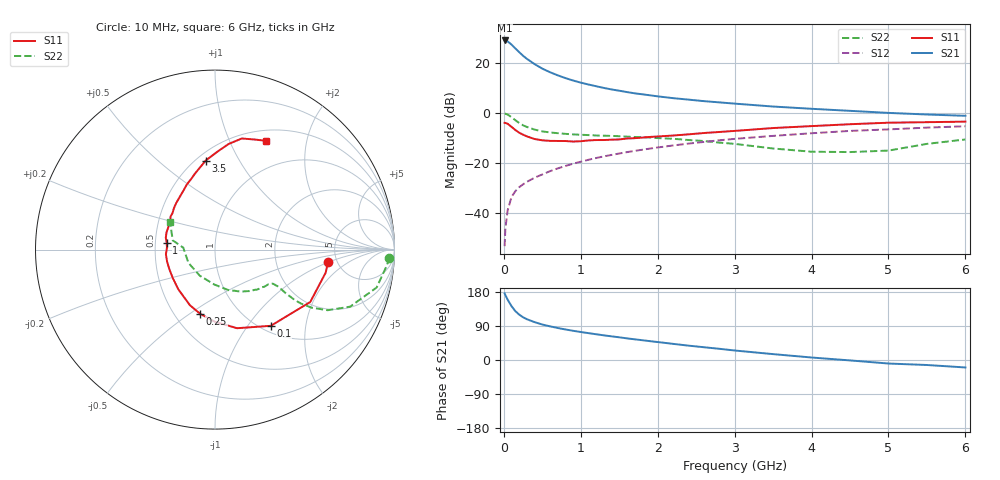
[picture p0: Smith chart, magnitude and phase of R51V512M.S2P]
! SIEMENS Small Signal Semiconductors
! BFR183
! Si NPN RF Bipolar Junction Transistor in SOT23
! VCE = 1.5 V  IC = 12 mA
! Common Emitter S-Parameters:  May  1996
# GHz  S  MA  R  50
!  f  S11  S21  S12  S22
! GHz  MAG  ANG  MAG  ANG  MAG  ANG  MAG  ANG
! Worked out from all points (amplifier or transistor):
!   36 points, 10 MHz to 6 GHz, reference 50 ohm
!   highest |S21| = 28.9 dB at 10 MHz (marker M1)
!   |S21| within 3 dB of that: start of sweep to 143.7 MHz
!   unconditionally stable (mu >= 1): 675.4 MHz to 2.536 GHz
!   at 250 MHz: K = 0.69, MSG = 25.6 dB, |S12| = -28.5 dB
!   at 1.4 GHz: K = 1.06, MAG = 11.6 dB, |S12| = -16.8 dB
!   at 6 GHz: K = 0.91, MSG = 2.1 dB, |S12| = -5.3 dB
!   S11 on the Smith chart (normalised r, x): 10 MHz: 4.22, -0.98; 100 MHz: 1.10, -1.30; 250 MHz: 0.67, -0.55; 1 GHz: 0.57, +0.05; 3.5 GHz: 0.56, +0.73; 6 GHz: 0.63, +1.37
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0.01  0.6338 -6.3  27.78 175.7  0.0022 88.6  0.9732 -2.6
0.02  0.6298 -11.8  27.59 171.2  0.005 80.5  0.9607 -5.4
0.05  0.6057 -28.8  26.59 159.0  0.0115 77.0  0.9251 -13.2
0.1  0.5263 -53.8  22.97 142.1  0.0211 70.2  0.8171 -22.9
0.15  0.455 -74.3  19.24 128.8  0.0275 65.3  0.7124 -28.3
0.2  0.402 -90.0  16.22 119.7  0.033 63.5  0.6283 -31.0
0.25  0.3676 -102.9  13.76 112.8  0.0376 62.4  0.5652 -32.1
0.3  0.3398 -114.3  11.94 107.6  0.0422 63.3  0.5237 -32.3
0.4  0.3013 -132.6  9.375 99.9  0.051 64.0  0.4641 -31.7
0.5  0.2836 -146.0  7.627 93.6  0.0592 65.1  0.4272 -30.8
0.6  0.2768 -156.5  6.464 88.8  0.0688 65.9  0.4073 -30.4
0.7  0.2753 -166.2  5.607 84.5  0.078 66.1  0.3935 -30.4
0.8  0.2746 -174.7  4.937 80.6  0.0874 66.2  0.3819 -30.4
1  0.272 171.7  4.007 73.9  0.1061 66.0  0.3667 -31.3
1.1  0.2819 166.5  3.678 70.9  0.1161 65.9  0.3604 -32.4
1.3  0.2874 156.0  3.142 65.1  0.1357 64.5  0.3505 -34.3
1.6  0.3083 143.5  2.599 57.1  0.1649 62.2  0.3358 -38.6
2.2  0.3533 123.8  1.966 42.6  0.224 56.7  0.3043 -49.4
3.5  0.4985 96.0  1.338 15.5  0.3476 40.6  0.1948 -91.0
4.5  0.5939 82.6  1.098 -1.1  0.437 27.8  0.1654 -153.3
5.5  0.6521 70.1  0.928 -13.2  0.5081 15.8  0.2409 167.7
6  0.6689 65.0  0.874 -19.7  0.541 8.1  0.2951 148.1
